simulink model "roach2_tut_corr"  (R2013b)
settings: Solver=VariableStepDiscrete  SolverMode=SingleTasking  StartTime=0.0  StopTime=100  RelTol=1e-3
undefined symbols (not defined in the file): add_latency, addr_width, Bit, bitfield, BitWidth, bram_latency, burst_size, casper_library_scopes, conv_latency, data_width, DelayLen, fan_latency, FFTSize, FFTStage, getfield, increment, led, Location, Lower, mult_latency, mux_latency, n_bits, n_bits_data, n_inputs, n_streams, n_taps, neg_latency, negate_latency, nsamples, pfb_size, pulse_len, reset_period, ROACH, ROACH2, snapshot, sx475t, sync_period, sync_period_bits, Upper, UseCounter, Width
libraries: xbsIndex_r4 x24444, casper_library_misc x73, xbsReplacements_r4 x34, casper_library_delays x14, xps_library x7
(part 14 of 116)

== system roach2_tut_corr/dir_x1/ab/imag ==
  addr : Inport
  data_in : Inport  Port=2
  we : Inport  Port=3
  calc_add : Subsystem
  convert_addr : xbsIndex_r4/Convert  gui_display_data_type=Fixed-point  arith_type=Unsigned  n_bits=addr_width  bin_pt=0  float_type=Single  exp_bits=8  fraction_bits=24  quantization=Truncate  overflow=Wrap  en=off  latency=0  dbl_ovrd=off  pipeline=off  block_type=convert
  convert_din1 : xbsIndex_r4/Convert  gui_display_data_type=Fixed-point  arith_type=Unsigned  n_bits=32  bin_pt=0  float_type=Single  exp_bits=8  fraction_bits=24  quantization=Truncate  overflow=Wrap  en=off  latency=0  dbl_ovrd=off  pipeline=off  block_type=convert
  convert_we : xbsIndex_r4/Convert  gui_display_data_type=Fixed-point  arith_type=Unsigned  n_bits=1  bin_pt=0  float_type=Single  exp_bits=8  fraction_bits=24  quantization=Truncate  overflow=Wrap  en=off  latency=0  dbl_ovrd=off  pipeline=off  block_type=convert
  mem : Subsystem
  munge_in : Subsystem  AncestorBlock=casper_library_flow_control/munge
  munge_out : Subsystem  AncestorBlock=casper_library_flow_control/munge
  roach2_tut_corr_dir_x1_ab_imag_addr : xbsIndex_r4/Gateway Out  inherit_from_input=off  hdl_port=on  timing_constraint=None  locs_specified=off  LOCs={'A5','B9','A9','C1','A3','G6','E9','A6','A7','A8','B8','B1','B3','D9','B5','B4','B6','C2'}  UseAsDAC=off  DACChannel='1'  block_type=gatewayout
  roach2_tut_corr_dir_x1_ab_imag_data_in : xbsIndex_r4/Gateway Out  inherit_from_input=off  hdl_port=on  timing_constraint=None  locs_specified=off  LOCs={'B21','B22','A22','B23','B19','C19','A20','A21','A23','B24','A24','A25','E18','D18','C18','B18'}  UseAsDAC=off  DACChannel='1'  block_type=gatewayout
  roach2_tut_corr_dir_x1_ab_imag_data_out : xbsIndex_r4/Gateway In  gui_display_data_type=Fixed-point  arith_type=Unsigned  n_bits=32  bin_pt=0  preci_type=Single  exp_width=8  frac_width=24  quantization=Truncate  overflow=Wrap  period=sample_rate  dbl_ovrd=off  timing_constraint=None  locs_specified=off  LOCs={}  UseAsADC=off  ADCChannel='1'  inherit_from_input=off  hdl_port=on  block_type=gatewayin
  roach2_tut_corr_dir_x1_ab_imag_we : xbsIndex_r4/Gateway Out  inherit_from_input=off  hdl_port=on  timing_constraint=None  locs_specified=off  LOCs={'A14'}  UseAsDAC=off  DACChannel='1'  block_type=gatewayout
  data_out : Outport
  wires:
  convert_addr/1 -> roach2_tut_corr_dir_x1_ab_imag_addr/1
  convert_din1/1 -> roach2_tut_corr_dir_x1_ab_imag_data_in/1
  data_in/1 -> munge_in/1(din)
  calc_add/1(out) -> convert_addr/1
  roach2_tut_corr_dir_x1_ab_imag_we/1 -> mem/3(In3)
  roach2_tut_corr_dir_x1_ab_imag_data_in/1 -> mem/2(In2)
  roach2_tut_corr_dir_x1_ab_imag_addr/1 -> mem/1(In1)
  convert_we/1 -> roach2_tut_corr_dir_x1_ab_imag_we/1
  roach2_tut_corr_dir_x1_ab_imag_data_out/1 -> munge_out/1(din)
  mem/1(Out1) -> roach2_tut_corr_dir_x1_ab_imag_data_out/1
  addr/1 -> calc_add/1(in)
  we/1 -> convert_we/1
  munge_out/1(dout) -> data_out/1
  munge_in/1(dout) -> convert_din1/1

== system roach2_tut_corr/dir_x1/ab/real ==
  addr : Inport
  data_in : Inport  Port=2
  we : Inport  Port=3
  calc_add : Subsystem
  convert_addr : xbsIndex_r4/Convert  gui_display_data_type=Fixed-point  arith_type=Unsigned  n_bits=addr_width  bin_pt=0  float_type=Single  exp_bits=8  fraction_bits=24  quantization=Truncate  overflow=Wrap  en=off  latency=0  dbl_ovrd=off  pipeline=off  block_type=convert
  convert_din1 : xbsIndex_r4/Convert  gui_display_data_type=Fixed-point  arith_type=Unsigned  n_bits=32  bin_pt=0  float_type=Single  exp_bits=8  fraction_bits=24  quantization=Truncate  overflow=Wrap  en=off  latency=0  dbl_ovrd=off  pipeline=off  block_type=convert
  convert_we : xbsIndex_r4/Convert  gui_display_data_type=Fixed-point  arith_type=Unsigned  n_bits=1  bin_pt=0  float_type=Single  exp_bits=8  fraction_bits=24  quantization=Truncate  overflow=Wrap  en=off  latency=0  dbl_ovrd=off  pipeline=off  block_type=convert
  mem : Subsystem
  munge_in : Subsystem  AncestorBlock=casper_library_flow_control/munge
  munge_out : Subsystem  AncestorBlock=casper_library_flow_control/munge
  roach2_tut_corr_dir_x1_ab_real_addr : xbsIndex_r4/Gateway Out  inherit_from_input=off  hdl_port=on  timing_constraint=None  locs_specified=off  LOCs={'A5','B9','A9','C1','A3','G6','E9','A6','A7','A8','B8','B1','B3','D9','B5','B4','B6','C2'}  UseAsDAC=off  DACChannel='1'  block_type=gatewayout
  roach2_tut_corr_dir_x1_ab_real_data_in : xbsIndex_r4/Gateway Out  inherit_from_input=off  hdl_port=on  timing_constraint=None  locs_specified=off  LOCs={'B21','B22','A22','B23','B19','C19','A20','A21','A23','B24','A24','A25','E18','D18','C18','B18'}  UseAsDAC=off  DACChannel='1'  block_type=gatewayout
  roach2_tut_corr_dir_x1_ab_real_data_out : xbsIndex_r4/Gateway In  gui_display_data_type=Fixed-point  arith_type=Unsigned  n_bits=32  bin_pt=0  preci_type=Single  exp_width=8  frac_width=24  quantization=Truncate  overflow=Wrap  period=sample_rate  dbl_ovrd=off  timing_constraint=None  locs_specified=off  LOCs={}  UseAsADC=off  ADCChannel='1'  inherit_from_input=off  hdl_port=on  block_type=gatewayin
  roach2_tut_corr_dir_x1_ab_real_we : xbsIndex_r4/Gateway Out  inherit_from_input=off  hdl_port=on  timing_constraint=None  locs_specified=off  LOCs={'A14'}  UseAsDAC=off  DACChannel='1'  block_type=gatewayout
  data_out : Outport
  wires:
  convert_addr/1 -> roach2_tut_corr_dir_x1_ab_real_addr/1
  convert_din1/1 -> roach2_tut_corr_dir_x1_ab_real_data_in/1
  data_in/1 -> munge_in/1(din)
  calc_add/1(out) -> convert_addr/1
  roach2_tut_corr_dir_x1_ab_real_we/1 -> mem/3(In3)
  roach2_tut_corr_dir_x1_ab_real_data_in/1 -> mem/2(In2)
  roach2_tut_corr_dir_x1_ab_real_addr/1 -> mem/1(In1)
  convert_we/1 -> roach2_tut_corr_dir_x1_ab_real_we/1
  roach2_tut_corr_dir_x1_ab_real_data_out/1 -> munge_out/1(din)
  mem/1(Out1) -> roach2_tut_corr_dir_x1_ab_real_data_out/1
  addr/1 -> calc_add/1(in)
  we/1 -> convert_we/1
  munge_out/1(dout) -> data_out/1
  munge_in/1(dout) -> convert_din1/1

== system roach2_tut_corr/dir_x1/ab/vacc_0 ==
  din : Inport
  new_acc : Inport  Port=2
  Adder0 : xbsIndex_r4/AddSub  mode=Addition  use_carryin=off  use_carryout=off  en=off  latency=2  precision=User Defined  arith_type="Signed  (2's comp)"  n_bits=32  bin_pt=6  quantization=Truncate  overflow=Wrap  dbl_ovrd=off  use_behavioral_HDL=on  hw_selection=Fabric  pipelined=off  use_rpm=on  block_type=addsub
  Mux0 : xbsIndex_r4/Mux  inputs=2  en=off  latency=0  precision=Full  arith_type="Signed  (2's comp)"  n_bits=8  bin_pt=2  quantization=Truncate  overflow=Wrap  dbl_ovrd=off  block_type=mux
  delay_bram : Subsystem
  pulse_ext : Subsystem
  warn period Adder00 : xbsReplacements_r4/Warning  period=1
  zero : xbsIndex_r4/Constant  const=0  gui_display_data_type=Fixed-point  arith_type=Signed (2's comp)  n_bits=32  bin_pt=6  preci_type=Single  exp_width=8  frac_width=24  explicit_period=on  period=1  equ=P=C  opselect=C  inp2=PCIN>>17  opr=+  inp1=P  carry=CIN  dbl_ovrd=off  block_type=constant
  dout : Outport
  valid : Outport  Port=2
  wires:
  delay_bram/1(Out1) -> Mux0/2, dout/1
  Adder0/1 -> delay_bram/1(In1)
  new_acc/1 -> pulse_ext/1(in)
  din/1 -> Adder0/1
  pulse_ext/1(out) -> valid/1, Mux0/1
  Mux0/1 -> Adder0/2
  zero/1 -> Mux0/3

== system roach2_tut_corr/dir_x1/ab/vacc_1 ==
  din : Inport
  new_acc : Inport  Port=2
  Adder0 : xbsIndex_r4/AddSub  mode=Addition  use_carryin=off  use_carryout=off  en=off  latency=2  precision=User Defined  arith_type="Signed  (2's comp)"  n_bits=32  bin_pt=6  quantization=Truncate  overflow=Wrap  dbl_ovrd=off  use_behavioral_HDL=on  hw_selection=Fabric  pipelined=off  use_rpm=on  block_type=addsub
  Mux0 : xbsIndex_r4/Mux  inputs=2  en=off  latency=0  precision=Full  arith_type="Signed  (2's comp)"  n_bits=8  bin_pt=2  quantization=Truncate  overflow=Wrap  dbl_ovrd=off  block_type=mux
  delay_bram : Subsystem
  pulse_ext : Subsystem
  warn period Adder00 : xbsReplacements_r4/Warning  period=1
  zero : xbsIndex_r4/Constant  const=0  gui_display_data_type=Fixed-point  arith_type=Signed (2's comp)  n_bits=32  bin_pt=6  preci_type=Single  exp_width=8  frac_width=24  explicit_period=on  period=1  equ=P=C  opselect=C  inp2=PCIN>>17  opr=+  inp1=P  carry=CIN  dbl_ovrd=off  block_type=constant
  dout : Outport
  valid : Outport  Port=2
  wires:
  zero/1 -> Mux0/3
  Mux0/1 -> Adder0/2
  pulse_ext/1(out) -> Mux0/1, valid/1
  din/1 -> Adder0/1
  new_acc/1 -> pulse_ext/1(in)
  Adder0/1 -> delay_bram/1(In1)
  delay_bram/1(Out1) -> dout/1, Mux0/2

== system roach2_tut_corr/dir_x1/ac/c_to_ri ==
  c : Inport
  force_im : xbsIndex_r4/Reinterpret  force_arith_type=on  arith_type="Signed  (2's comp)"  force_bin_pt=on  bin_pt=bin_pt  block_type=reinterpret
  force_re : xbsIndex_r4/Reinterpret  force_arith_type=on  arith_type="Signed  (2's comp)"  force_bin_pt=on  bin_pt=bin_pt  block_type=reinterpret
  slice_im : xbsIndex_r4/Slice  nbits=n_bits  boolean_output=off  mode=Lower Bit Location + Width  bit1=0  base1=MSB of Input  bit0=0  base0=LSB of Input  dbl_ovrd=off  block_type=slice
  slice_re : xbsIndex_r4/Slice  nbits=n_bits  boolean_output=off  mode=Upper Bit Location + Width  bit1=0  base1=MSB of Input  bit0=0  base0=LSB of Input  dbl_ovrd=off  block_type=slice
  re : Outport
  im : Outport  Port=2
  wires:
  c/1 -> slice_im/1, slice_re/1
  force_im/1 -> im/1
  force_re/1 -> re/1
  slice_im/1 -> force_im/1
  slice_re/1 -> force_re/1

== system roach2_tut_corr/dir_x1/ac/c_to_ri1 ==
  c : Inport
  force_im : xbsIndex_r4/Reinterpret  force_arith_type=on  arith_type="Signed  (2's comp)"  force_bin_pt=on  bin_pt=bin_pt  block_type=reinterpret
  force_re : xbsIndex_r4/Reinterpret  force_arith_type=on  arith_type="Signed  (2's comp)"  force_bin_pt=on  bin_pt=bin_pt  block_type=reinterpret
  slice_im : xbsIndex_r4/Slice  nbits=n_bits  boolean_output=off  mode=Lower Bit Location + Width  bit1=0  base1=MSB of Input  bit0=0  base0=LSB of Input  dbl_ovrd=off  block_type=slice
  slice_re : xbsIndex_r4/Slice  nbits=n_bits  boolean_output=off  mode=Upper Bit Location + Width  bit1=0  base1=MSB of Input  bit0=0  base0=LSB of Input  dbl_ovrd=off  block_type=slice
  re : Outport
  im : Outport  Port=2
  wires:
  c/1 -> slice_im/1, slice_re/1
  force_im/1 -> im/1
  force_re/1 -> re/1
  slice_im/1 -> force_im/1
  slice_re/1 -> force_re/1

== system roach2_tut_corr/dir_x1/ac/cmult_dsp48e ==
  a_re : Inport
  a_im : Inport  Port=2
  b_re : Inport  Port=3
  b_im : Inport  Port=4
  Convert{,1..2,5} (4 alike) : xbsIndex_r4/Convert  gui_display_data_type=Fixed-point  arith_type="Signed  (2's comp)"  n_bits=30  bin_pt=0  float_type=Single  exp_bits=8  fraction_bits=24  quantization=Truncate  overflow=Wrap  en=off  latency=0  dbl_ovrd=off  pipeline=on  block_type=convert
  Convert{3..4,6..7} (4 alike) : xbsIndex_r4/Convert  gui_display_data_type=Fixed-point  arith_type="Signed  (2's comp)"  n_bits=18  bin_pt=0  float_type=Single  exp_bits=8  fraction_bits=24  quantization=Truncate  overflow=Wrap  en=off  latency=0  dbl_ovrd=off  pipeline=on  block_type=convert
  DSP48E_0 : xbsIndex_r4/DSP48E  use_a=Direct from A Port  use_b=Direct from B Port  reset_preg=off  pattern_from_creg=off  pattern='000000000000'  mask_from_creg=off  pattern_mask='3FFFFFFFFFFF'  sel_rounding_mask=Select mask  use_op=off  use_creg=off  rst_all=off  en_all=off  use_pcin=off  use_carrycascin=off  use_multsignin=off  use_carryout=off  use_patterndetect=off  use_patternbdetect=off  use_overflow=off  use_underflow=off  use_acout=off  use_bcout=off  use_pcout=on  use_multsignout=off  use_carrycascout=off  pipeline_a=1  pipeline_b=1  pipeline_acout=1  pipeline_bcout=1  pipeline_c=on  pipeline_p=on  pipeline_mult=on  pipeline_opmode=on  pipeline_alumode=on  pipeline_carryin=on  pipeline_carryinsel=on  rst_a=off  rst_b=off  rst_c=off  rst_mult=off  rst_p=off  rst_carry_in=off  rst_alumode=off  rst_ctrl=off  en_a1=off  en_a2=off  en_b1=off  en_b2=off  en_c=off  en_mult=off  en_p=off  en_carry_in=off  en_alumode=off  en_multcarryin=off  en_ctrl=off  use_synth_model=off  addsub_mode=ONE48  xl_useadderonly=off  block_type=dsp48e
  DSP48E_1 : xbsIndex_r4/DSP48E  use_a=Direct from A Port  use_b=Direct from B Port  reset_preg=off  pattern_from_creg=off  pattern='000000000000'  mask_from_creg=off  pattern_mask='3FFFFFFFFFFF'  sel_rounding_mask=Select mask  use_op=off  use_creg=off  rst_all=off  en_all=off  use_pcin=on  use_carrycascin=off  use_multsignin=off  use_carryout=off  use_patterndetect=off  use_patternbdetect=off  use_overflow=off  use_underflow=off  use_acout=off  use_bcout=off  use_pcout=off  use_multsignout=off  use_carrycascout=off  pipeline_a=2  pipeline_b=2  pipeline_acout=1  pipeline_bcout=1  pipeline_c=on  pipeline_p=on  pipeline_mult=on  pipeline_opmode=on  pipeline_alumode=on  pipeline_carryin=on  pipeline_carryinsel=on  rst_a=off  rst_b=off  rst_c=off  rst_mult=off  rst_p=off  rst_carry_in=off  rst_alumode=off  rst_ctrl=off  en_a1=off  en_a2=off  en_b1=off  en_b2=off  en_c=off  en_mult=off  en_p=off  en_carry_in=off  en_alumode=off  en_multcarryin=off  en_ctrl=off  use_synth_model=off  addsub_mode=ONE48  xl_useadderonly=off  block_type=dsp48e
  DSP48E_2 : xbsIndex_r4/DSP48E  use_a=Direct from A Port  use_b=Direct from B Port  reset_preg=off  pattern_from_creg=off  pattern='000000000000'  mask_from_creg=off  pattern_mask='3FFFFFFFFFFF'  sel_rounding_mask=Select mask  use_op=off  use_creg=off  rst_all=off  en_all=off  use_pcin=off  use_carrycascin=off  use_multsignin=off  use_carryout=off  use_patterndetect=off  use_patternbdetect=off  use_overflow=off  use_underflow=off  use_acout=off  use_bcout=off  use_pcout=on  use_multsignout=off  use_carrycascout=off  pipeline_a=1  pipeline_b=1  pipeline_acout=1  pipeline_bcout=1  pipeline_c=on  pipeline_p=on  pipeline_mult=on  pipeline_opmode=on  pipeline_alumode=on  pipeline_carryin=on  pipeline_carryinsel=on  rst_a=off  rst_b=off  rst_c=off  rst_mult=off  rst_p=off  rst_carry_in=off  rst_alumode=off  rst_ctrl=off  en_a1=off  en_a2=off  en_b1=off  en_b2=off  en_c=off  en_mult=off  en_p=off  en_carry_in=off  en_alumode=off  en_multcarryin=off  en_ctrl=off  use_synth_model=off  addsub_mode=ONE48  xl_useadderonly=off  block_type=dsp48e
  DSP48E_3 : xbsIndex_r4/DSP48E  use_a=Direct from A Port  use_b=Direct from B Port  reset_preg=off  pattern_from_creg=off  pattern='000000000000'  mask_from_creg=off  pattern_mask='3FFFFFFFFFFF'  sel_rounding_mask=Select mask  use_op=off  use_creg=off  rst_all=off  en_all=off  use_pcin=on  use_carrycascin=off  use_multsignin=off  use_carryout=off  use_patterndetect=off  use_patternbdetect=off  use_overflow=off  use_underflow=off  use_acout=off  use_bcout=off  use_pcout=off  use_multsignout=off  use_carrycascout=off  pipeline_a=2  pipeline_b=2  pipeline_acout=1  pipeline_bcout=1  pipeline_c=on  pipeline_p=on  pipeline_mult=on  pipeline_opmode=on  pipeline_alumode=on  pipeline_carryin=on  pipeline_carryinsel=on  rst_a=off  rst_b=off  rst_c=off  rst_mult=off  rst_p=off  rst_carry_in=off  rst_alumode=off  rst_ctrl=off  en_a1=off  en_a2=off  en_b1=off  en_b2=off  en_c=off  en_mult=off  en_p=off  en_carry_in=off  en_alumode=off  en_multcarryin=off  en_ctrl=off  use_synth_model=off  addsub_mode=ONE48  xl_useadderonly=off  block_type=dsp48e
  Terminator : Terminator
  Terminator1 : Terminator
  alumode0 : xbsIndex_r4/Constant  const=3  gui_display_data_type=Fixed-point  arith_type=Unsigned  n_bits=4  bin_pt=0  preci_type=Single  exp_width=8  frac_width=24  explicit_period=off  period=1  equ=P=C  opselect=C  inp2=PCIN>>17  opr=+  inp1=P  carry=CIN  dbl_ovrd=off  block_type=constant
  alumode1 : xbsIndex_r4/Constant  const=0  gui_display_data_type=Fixed-point  arith_type=Unsigned  n_bits=4  bin_pt=0  preci_type=Single  exp_width=8  frac_width=24  explicit_period=off  period=1  equ=P=C  opselect=C  inp2=PCIN>>17  opr=+  inp1=P  carry=CIN  dbl_ovrd=off  block_type=constant
  alumode2 : xbsIndex_r4/Constant  const=0  gui_display_data_type=Fixed-point  arith_type=Unsigned  n_bits=4  bin_pt=0  preci_type=Single  exp_width=8  frac_width=24  explicit_period=off  period=1  equ=P=C  opselect=C  inp2=PCIN>>17  opr=+  inp1=P  carry=CIN  dbl_ovrd=off  block_type=constant
  alumode3 : xbsIndex_r4/Constant  const=0  gui_display_data_type=Fixed-point  arith_type=Unsigned  n_bits=4  bin_pt=0  preci_type=Single  exp_width=8  frac_width=24  explicit_period=off  period=1  equ=P=C  opselect=C  inp2=PCIN>>17  opr=+  inp1=P  carry=CIN  dbl_ovrd=off  block_type=constant
  carryin{0..3} (4 alike) : xbsIndex_r4/Constant  const=0  gui_display_data_type=Fixed-point  arith_type=Unsigned  n_bits=1  bin_pt=0  preci_type=Single  exp_width=8  frac_width=24  explicit_period=off  period=1  equ=P=C  opselect=C  inp2=PCIN>>17  opr=+  inp1=P  carry=CIN  dbl_ovrd=off  block_type=constant
  carryinsel{0..3} (4 alike) : xbsIndex_r4/Constant  const=0  gui_display_data_type=Fixed-point  arith_type=Unsigned  n_bits=3  bin_pt=0  preci_type=Single  exp_width=8  frac_width=24  explicit_period=off  period=1  equ=P=C  opselect=C  inp2=PCIN>>17  opr=+  inp1=P  carry=CIN  dbl_ovrd=off  block_type=constant
  cast_c_im : xbsIndex_r4/Convert  gui_display_data_type=Fixed-point  arith_type="Signed  (2's comp)"  n_bits=9  bin_pt=6  float_type=Single  exp_bits=8  fraction_bits=24  quantization=Truncate  overflow=Wrap  en=off  latency=0  dbl_ovrd=off  pipeline=on  block_type=convert
  cast_c_re : xbsIndex_r4/Convert  gui_display_data_type=Fixed-point  arith_type="Signed  (2's comp)"  n_bits=9  bin_pt=6  float_type=Single  exp_bits=8  fraction_bits=24  quantization=Truncate  overflow=Wrap  en=off  latency=0  dbl_ovrd=off  pipeline=on  block_type=convert
  opmode0 : xbsIndex_r4/Constant  const=5  gui_display_data_type=Fixed-point  arith_type=Unsigned  n_bits=7  bin_pt=0  preci_type=Single  exp_width=8  frac_width=24  explicit_period=off  period=1  equ=P=C  opselect=C  inp2=PCIN>>17  opr=+  inp1=P  carry=CIN  dbl_ovrd=off  block_type=constant
  opmode1 : xbsIndex_r4/Constant  const=21  gui_display_data_type=Fixed-point  arith_type=Unsigned  n_bits=7  bin_pt=0  preci_type=Single  exp_width=8  frac_width=24  explicit_period=off  period=1  equ=P=C  opselect=C  inp2=PCIN>>17  opr=+  inp1=P  carry=CIN  dbl_ovrd=off  block_type=constant
  opmode2 : xbsIndex_r4/Constant  const=5  gui_display_data_type=Fixed-point  arith_type=Unsigned  n_bits=7  bin_pt=0  preci_type=Single  exp_width=8  frac_width=24  explicit_period=off  period=1  equ=P=C  opselect=C  inp2=PCIN>>17  opr=+  inp1=P  carry=CIN  dbl_ovrd=off  block_type=constant
  opmode3 : xbsIndex_r4/Constant  const=21  gui_display_data_type=Fixed-point  arith_type=Unsigned  n_bits=7  bin_pt=0  preci_type=Single  exp_width=8  frac_width=24  explicit_period=off  period=1  equ=P=C  opselect=C  inp2=PCIN>>17  opr=+  inp1=P  carry=CIN  dbl_ovrd=off  block_type=constant
  realign_a_im : xbsIndex_r4/Convert  gui_display_data_type=Fixed-point  arith_type="Signed  (2's comp)"  n_bits=4  bin_pt=3  float_type=Single  exp_bits=8  fraction_bits=24  quantization=Truncate  overflow=Wrap  en=off  latency=0  dbl_ovrd=off  pipeline=on  block_type=convert
  realign_a_re : xbsIndex_r4/Convert  gui_display_data_type=Fixed-point  arith_type="Signed  (2's comp)"  n_bits=4  bin_pt=3  float_type=Single  exp_bits=8  fraction_bits=24  quantization=Truncate  overflow=Wrap  en=off  latency=0  dbl_ovrd=off  pipeline=on  block_type=convert
  realign_b_im : xbsIndex_r4/Convert  gui_display_data_type=Fixed-point  arith_type="Signed  (2's comp)"  n_bits=4  bin_pt=3  float_type=Single  exp_bits=8  fraction_bits=24  quantization=Truncate  overflow=Wrap  en=off  latency=0  dbl_ovrd=off  pipeline=on  block_type=convert
  realign_b_re : xbsIndex_r4/Convert  gui_display_data_type=Fixed-point  arith_type="Signed  (2's comp)"  n_bits=4  bin_pt=3  float_type=Single  exp_bits=8  fraction_bits=24  quantization=Truncate  overflow=Wrap  en=off  latency=0  dbl_ovrd=off  pipeline=on  block_type=convert
  reinterp_a_im : xbsIndex_r4/Reinterpret  force_arith_type=on  arith_type="Signed  (2's comp)"  force_bin_pt=on  bin_pt=0  block_type=reinterpret
  reinterp_a_re : xbsIndex_r4/Reinterpret  force_arith_type=on  arith_type="Signed  (2's comp)"  force_bin_pt=on  bin_pt=0  block_type=reinterpret
  reinterp_b_im : xbsIndex_r4/Reinterpret  force_arith_type=on  arith_type="Signed  (2's comp)"  force_bin_pt=on  bin_pt=0  block_type=reinterpret
  reinterp_b_re : xbsIndex_r4/Reinterpret  force_arith_type=on  arith_type="Signed  (2's comp)"  force_bin_pt=on  bin_pt=0  block_type=reinterpret
  reinterp_c_im : xbsIndex_r4/Reinterpret  force_arith_type=on  arith_type="Signed  (2's comp)"  force_bin_pt=on  bin_pt=6  block_type=reinterpret
  reinterp_c_re : xbsIndex_r4/Reinterpret  force_arith_type=on  arith_type="Signed  (2's comp)"  force_bin_pt=on  bin_pt=6  block_type=reinterpret
  c_re : Outport
  c_im : Outport  Port=2
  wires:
  b_im/1 -> realign_b_im/1
  b_re/1 -> realign_b_re/1
  a_im/1 -> realign_a_im/1
  a_re/1 -> realign_a_re/1
  cast_c_im/1 -> c_im/1
  cast_c_re/1 -> c_re/1
  reinterp_b_im/1 -> Convert3/1, Convert7/1
  reinterp_b_re/1 -> Convert6/1, Convert4/1
  reinterp_a_im/1 -> Convert/1, Convert1/1
  reinterp_a_re/1 -> Convert5/1, Convert2/1
  realign_b_im/1 -> reinterp_b_im/1
  realign_b_re/1 -> reinterp_b_re/1
  realign_a_im/1 -> reinterp_a_im/1
  realign_a_re/1 -> reinterp_a_re/1
  Convert/1 -> DSP48E_3/1
  DSP48E_2/1 -> Terminator/1
  DSP48E_2/2 -> DSP48E_3/3
  opmode3/1 -> DSP48E_3/4
  alumode3/1 -> DSP48E_3/5
  carryin3/1 -> DSP48E_3/6
  carryinsel3/1 -> DSP48E_3/7
  Convert3/1 -> DSP48E_3/2
  Convert2/1 -> DSP48E_2/1
  Convert4/1 -> DSP48E_2/2
  opmode2/1 -> DSP48E_2/3
  alumode2/1 -> DSP48E_2/4
  carryin2/1 -> DSP48E_2/5
  carryinsel2/1 -> DSP48E_2/6
  reinterp_c_re/1 -> cast_c_re/1
  DSP48E_3/1 -> reinterp_c_re/1
  Convert1/1 -> DSP48E_1/1
  DSP48E_0/1 -> Terminator1/1
  DSP48E_0/2 -> DSP48E_1/3
  opmode1/1 -> DSP48E_1/4
  alumode1/1 -> DSP48E_1/5
  carryin1/1 -> DSP48E_1/6
  carryinsel1/1 -> DSP48E_1/7
  Convert6/1 -> DSP48E_1/2
  Convert5/1 -> DSP48E_0/1
  Convert7/1 -> DSP48E_0/2
  opmode0/1 -> DSP48E_0/3
  alumode0/1 -> DSP48E_0/4
  carryin0/1 -> DSP48E_0/5
  carryinsel0/1 -> DSP48E_0/6
  DSP48E_1/1 -> reinterp_c_im/1
  reinterp_c_im/1 -> cast_c_im/1

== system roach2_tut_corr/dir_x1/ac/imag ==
  addr : Inport
  data_in : Inport  Port=2
  we : Inport  Port=3
  calc_add : Subsystem
  convert_addr : xbsIndex_r4/Convert  gui_display_data_type=Fixed-point  arith_type=Unsigned  n_bits=addr_width  bin_pt=0  float_type=Single  exp_bits=8  fraction_bits=24  quantization=Truncate  overflow=Wrap  en=off  latency=0  dbl_ovrd=off  pipeline=off  block_type=convert
  convert_din1 : xbsIndex_r4/Convert  gui_display_data_type=Fixed-point  arith_type=Unsigned  n_bits=32  bin_pt=0  float_type=Single  exp_bits=8  fraction_bits=24  quantization=Truncate  overflow=Wrap  en=off  latency=0  dbl_ovrd=off  pipeline=off  block_type=convert
  convert_we : xbsIndex_r4/Convert  gui_display_data_type=Fixed-point  arith_type=Unsigned  n_bits=1  bin_pt=0  float_type=Single  exp_bits=8  fraction_bits=24  quantization=Truncate  overflow=Wrap  en=off  latency=0  dbl_ovrd=off  pipeline=off  block_type=convert
  mem : Subsystem
  munge_in : Subsystem  AncestorBlock=casper_library_flow_control/munge
  munge_out : Subsystem  AncestorBlock=casper_library_flow_control/munge
  roach2_tut_corr_dir_x1_ac_imag_addr : xbsIndex_r4/Gateway Out  inherit_from_input=off  hdl_port=on  timing_constraint=None  locs_specified=off  LOCs={'A5','B9','A9','C1','A3','G6','E9','A6','A7','A8','B8','B1','B3','D9','B5','B4','B6','C2'}  UseAsDAC=off  DACChannel='1'  block_type=gatewayout
  roach2_tut_corr_dir_x1_ac_imag_data_in : xbsIndex_r4/Gateway Out  inherit_from_input=off  hdl_port=on  timing_constraint=None  locs_specified=off  LOCs={'B21','B22','A22','B23','B19','C19','A20','A21','A23','B24','A24','A25','E18','D18','C18','B18'}  UseAsDAC=off  DACChannel='1'  block_type=gatewayout
  roach2_tut_corr_dir_x1_ac_imag_data_out : xbsIndex_r4/Gateway In  gui_display_data_type=Fixed-point  arith_type=Unsigned  n_bits=32  bin_pt=0  preci_type=Single  exp_width=8  frac_width=24  quantization=Truncate  overflow=Wrap  period=sample_rate  dbl_ovrd=off  timing_constraint=None  locs_specified=off  LOCs={}  UseAsADC=off  ADCChannel='1'  inherit_from_input=off  hdl_port=on  block_type=gatewayin
  roach2_tut_corr_dir_x1_ac_imag_we : xbsIndex_r4/Gateway Out  inherit_from_input=off  hdl_port=on  timing_constraint=None  locs_specified=off  LOCs={'A14'}  UseAsDAC=off  DACChannel='1'  block_type=gatewayout
  data_out : Outport
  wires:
  convert_addr/1 -> roach2_tut_corr_dir_x1_ac_imag_addr/1
  convert_din1/1 -> roach2_tut_corr_dir_x1_ac_imag_data_in/1
  data_in/1 -> munge_in/1(din)
  calc_add/1(out) -> convert_addr/1
  roach2_tut_corr_dir_x1_ac_imag_we/1 -> mem/3(In3)
  roach2_tut_corr_dir_x1_ac_imag_data_in/1 -> mem/2(In2)
  roach2_tut_corr_dir_x1_ac_imag_addr/1 -> mem/1(In1)
  convert_we/1 -> roach2_tut_corr_dir_x1_ac_imag_we/1
  roach2_tut_corr_dir_x1_ac_imag_data_out/1 -> munge_out/1(din)
  mem/1(Out1) -> roach2_tut_corr_dir_x1_ac_imag_data_out/1
  addr/1 -> calc_add/1(in)
  we/1 -> convert_we/1
  munge_out/1(dout) -> data_out/1
  munge_in/1(dout) -> convert_din1/1

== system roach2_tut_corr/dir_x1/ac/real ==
  addr : Inport
  data_in : Inport  Port=2
  we : Inport  Port=3
  calc_add : Subsystem
  convert_addr : xbsIndex_r4/Convert  gui_display_data_type=Fixed-point  arith_type=Unsigned  n_bits=addr_width  bin_pt=0  float_type=Single  exp_bits=8  fraction_bits=24  quantization=Truncate  overflow=Wrap  en=off  latency=0  dbl_ovrd=off  pipeline=off  block_type=convert
  convert_din1 : xbsIndex_r4/Convert  gui_display_data_type=Fixed-point  arith_type=Unsigned  n_bits=32  bin_pt=0  float_type=Single  exp_bits=8  fraction_bits=24  quantization=Truncate  overflow=Wrap  en=off  latency=0  dbl_ovrd=off  pipeline=off  block_type=convert
  convert_we : xbsIndex_r4/Convert  gui_display_data_type=Fixed-point  arith_type=Unsigned  n_bits=1  bin_pt=0  float_type=Single  exp_bits=8  fraction_bits=24  quantization=Truncate  overflow=Wrap  en=off  latency=0  dbl_ovrd=off  pipeline=off  block_type=convert
  mem : Subsystem
  munge_in : Subsystem  AncestorBlock=casper_library_flow_control/munge
  munge_out : Subsystem  AncestorBlock=casper_library_flow_control/munge
  roach2_tut_corr_dir_x1_ac_real_addr : xbsIndex_r4/Gateway Out  inherit_from_input=off  hdl_port=on  timing_constraint=None  locs_specified=off  LOCs={'A5','B9','A9','C1','A3','G6','E9','A6','A7','A8','B8','B1','B3','D9','B5','B4','B6','C2'}  UseAsDAC=off  DACChannel='1'  block_type=gatewayout
  roach2_tut_corr_dir_x1_ac_real_data_in : xbsIndex_r4/Gateway Out  inherit_from_input=off  hdl_port=on  timing_constraint=None  locs_specified=off  LOCs={'B21','B22','A22','B23','B19','C19','A20','A21','A23','B24','A24','A25','E18','D18','C18','B18'}  UseAsDAC=off  DACChannel='1'  block_type=gatewayout
  roach2_tut_corr_dir_x1_ac_real_data_out : xbsIndex_r4/Gateway In  gui_display_data_type=Fixed-point  arith_type=Unsigned  n_bits=32  bin_pt=0  preci_type=Single  exp_width=8  frac_width=24  quantization=Truncate  overflow=Wrap  period=sample_rate  dbl_ovrd=off  timing_constraint=None  locs_specified=off  LOCs={}  UseAsADC=off  ADCChannel='1'  inherit_from_input=off  hdl_port=on  block_type=gatewayin
  roach2_tut_corr_dir_x1_ac_real_we : xbsIndex_r4/Gateway Out  inherit_from_input=off  hdl_port=on  timing_constraint=None  locs_specified=off  LOCs={'A14'}  UseAsDAC=off  DACChannel='1'  block_type=gatewayout
  data_out : Outport
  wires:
  convert_addr/1 -> roach2_tut_corr_dir_x1_ac_real_addr/1
  convert_din1/1 -> roach2_tut_corr_dir_x1_ac_real_data_in/1
  data_in/1 -> munge_in/1(din)
  calc_add/1(out) -> convert_addr/1
  roach2_tut_corr_dir_x1_ac_real_we/1 -> mem/3(In3)
  roach2_tut_corr_dir_x1_ac_real_data_in/1 -> mem/2(In2)
  roach2_tut_corr_dir_x1_ac_real_addr/1 -> mem/1(In1)
  convert_we/1 -> roach2_tut_corr_dir_x1_ac_real_we/1
  roach2_tut_corr_dir_x1_ac_real_data_out/1 -> munge_out/1(din)
  mem/1(Out1) -> roach2_tut_corr_dir_x1_ac_real_data_out/1
  addr/1 -> calc_add/1(in)
  we/1 -> convert_we/1
  munge_out/1(dout) -> data_out/1
  munge_in/1(dout) -> convert_din1/1

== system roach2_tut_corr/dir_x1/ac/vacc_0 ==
  din : Inport
  new_acc : Inport  Port=2
  Adder0 : xbsIndex_r4/AddSub  mode=Addition  use_carryin=off  use_carryout=off  en=off  latency=2  precision=User Defined  arith_type="Signed  (2's comp)"  n_bits=32  bin_pt=6  quantization=Truncate  overflow=Wrap  dbl_ovrd=off  use_behavioral_HDL=on  hw_selection=Fabric  pipelined=off  use_rpm=on  block_type=addsub
  Mux0 : xbsIndex_r4/Mux  inputs=2  en=off  latency=0  precision=Full  arith_type="Signed  (2's comp)"  n_bits=8  bin_pt=2  quantization=Truncate  overflow=Wrap  dbl_ovrd=off  block_type=mux
  delay_bram : Subsystem
  pulse_ext : Subsystem
  warn period Adder00 : xbsReplacements_r4/Warning  period=1
  zero : xbsIndex_r4/Constant  const=0  gui_display_data_type=Fixed-point  arith_type=Signed (2's comp)  n_bits=32  bin_pt=6  preci_type=Single  exp_width=8  frac_width=24  explicit_period=on  period=1  equ=P=C  opselect=C  inp2=PCIN>>17  opr=+  inp1=P  carry=CIN  dbl_ovrd=off  block_type=constant
  dout : Outport
  valid : Outport  Port=2
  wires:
  zero/1 -> Mux0/3
  Mux0/1 -> Adder0/2
  pulse_ext/1(out) -> Mux0/1, valid/1
  din/1 -> Adder0/1
  new_acc/1 -> pulse_ext/1(in)
  Adder0/1 -> delay_bram/1(In1)
  delay_bram/1(Out1) -> dout/1, Mux0/2

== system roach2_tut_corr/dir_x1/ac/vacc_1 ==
  din : Inport
  new_acc : Inport  Port=2
  Adder0 : xbsIndex_r4/AddSub  mode=Addition  use_carryin=off  use_carryout=off  en=off  latency=2  precision=User Defined  arith_type="Signed  (2's comp)"  n_bits=32  bin_pt=6  quantization=Truncate  overflow=Wrap  dbl_ovrd=off  use_behavioral_HDL=on  hw_selection=Fabric  pipelined=off  use_rpm=on  block_type=addsub
  Mux0 : xbsIndex_r4/Mux  inputs=2  en=off  latency=0  precision=Full  arith_type="Signed  (2's comp)"  n_bits=8  bin_pt=2  quantization=Truncate  overflow=Wrap  dbl_ovrd=off  block_type=mux
  delay_bram : Subsystem
  pulse_ext : Subsystem
  warn period Adder00 : xbsReplacements_r4/Warning  period=1
  zero : xbsIndex_r4/Constant  const=0  gui_display_data_type=Fixed-point  arith_type=Signed (2's comp)  n_bits=32  bin_pt=6  preci_type=Single  exp_width=8  frac_width=24  explicit_period=on  period=1  equ=P=C  opselect=C  inp2=PCIN>>17  opr=+  inp1=P  carry=CIN  dbl_ovrd=off  block_type=constant
  dout : Outport
  valid : Outport  Port=2
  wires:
  delay_bram/1(Out1) -> Mux0/2, dout/1
  Adder0/1 -> delay_bram/1(In1)
  new_acc/1 -> pulse_ext/1(in)
  din/1 -> Adder0/1
  pulse_ext/1(out) -> valid/1, Mux0/1
  Mux0/1 -> Adder0/2
  zero/1 -> Mux0/3

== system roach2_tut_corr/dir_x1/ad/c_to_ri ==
  c : Inport
  force_im : xbsIndex_r4/Reinterpret  force_arith_type=on  arith_type="Signed  (2's comp)"  force_bin_pt=on  bin_pt=bin_pt  block_type=reinterpret
  force_re : xbsIndex_r4/Reinterpret  force_arith_type=on  arith_type="Signed  (2's comp)"  force_bin_pt=on  bin_pt=bin_pt  block_type=reinterpret
  slice_im : xbsIndex_r4/Slice  nbits=n_bits  boolean_output=off  mode=Lower Bit Location + Width  bit1=0  base1=MSB of Input  bit0=0  base0=LSB of Input  dbl_ovrd=off  block_type=slice
  slice_re : xbsIndex_r4/Slice  nbits=n_bits  boolean_output=off  mode=Upper Bit Location + Width  bit1=0  base1=MSB of Input  bit0=0  base0=LSB of Input  dbl_ovrd=off  block_type=slice
  re : Outport
  im : Outport  Port=2
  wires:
  slice_re/1 -> force_re/1
  slice_im/1 -> force_im/1
  force_re/1 -> re/1
  force_im/1 -> im/1
  c/1 -> slice_re/1, slice_im/1

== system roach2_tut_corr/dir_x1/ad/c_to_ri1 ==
  c : Inport
  force_im : xbsIndex_r4/Reinterpret  force_arith_type=on  arith_type="Signed  (2's comp)"  force_bin_pt=on  bin_pt=bin_pt  block_type=reinterpret
  force_re : xbsIndex_r4/Reinterpret  force_arith_type=on  arith_type="Signed  (2's comp)"  force_bin_pt=on  bin_pt=bin_pt  block_type=reinterpret
  slice_im : xbsIndex_r4/Slice  nbits=n_bits  boolean_output=off  mode=Lower Bit Location + Width  bit1=0  base1=MSB of Input  bit0=0  base0=LSB of Input  dbl_ovrd=off  block_type=slice
  slice_re : xbsIndex_r4/Slice  nbits=n_bits  boolean_output=off  mode=Upper Bit Location + Width  bit1=0  base1=MSB of Input  bit0=0  base0=LSB of Input  dbl_ovrd=off  block_type=slice
  re : Outport
  im : Outport  Port=2
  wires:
  slice_re/1 -> force_re/1
  slice_im/1 -> force_im/1
  force_re/1 -> re/1
  force_im/1 -> im/1
  c/1 -> slice_re/1, slice_im/1

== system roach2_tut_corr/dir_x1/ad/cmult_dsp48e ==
  a_re : Inport
  a_im : Inport  Port=2
  b_re : Inport  Port=3
  b_im : Inport  Port=4
  Convert{,1..2,5} (4 alike) : xbsIndex_r4/Convert  gui_display_data_type=Fixed-point  arith_type="Signed  (2's comp)"  n_bits=30  bin_pt=0  float_type=Single  exp_bits=8  fraction_bits=24  quantization=Truncate  overflow=Wrap  en=off  latency=0  dbl_ovrd=off  pipeline=on  block_type=convert
  Convert{3..4,6..7} (4 alike) : xbsIndex_r4/Convert  gui_display_data_type=Fixed-point  arith_type="Signed  (2's comp)"  n_bits=18  bin_pt=0  float_type=Single  exp_bits=8  fraction_bits=24  quantization=Truncate  overflow=Wrap  en=off  latency=0  dbl_ovrd=off  pipeline=on  block_type=convert
  DSP48E_0 : xbsIndex_r4/DSP48E  use_a=Direct from A Port  use_b=Direct from B Port  reset_preg=off  pattern_from_creg=off  pattern='000000000000'  mask_from_creg=off  pattern_mask='3FFFFFFFFFFF'  sel_rounding_mask=Select mask  use_op=off  use_creg=off  rst_all=off  en_all=off  use_pcin=off  use_carrycascin=off  use_multsignin=off  use_carryout=off  use_patterndetect=off  use_patternbdetect=off  use_overflow=off  use_underflow=off  use_acout=off  use_bcout=off  use_pcout=on  use_multsignout=off  use_carrycascout=off  pipeline_a=1  pipeline_b=1  pipeline_acout=1  pipeline_bcout=1  pipeline_c=on  pipeline_p=on  pipeline_mult=on  pipeline_opmode=on  pipeline_alumode=on  pipeline_carryin=on  pipeline_carryinsel=on  rst_a=off  rst_b=off  rst_c=off  rst_mult=off  rst_p=off  rst_carry_in=off  rst_alumode=off  rst_ctrl=off  en_a1=off  en_a2=off  en_b1=off  en_b2=off  en_c=off  en_mult=off  en_p=off  en_carry_in=off  en_alumode=off  en_multcarryin=off  en_ctrl=off  use_synth_model=off  addsub_mode=ONE48  xl_useadderonly=off  block_type=dsp48e
  DSP48E_1 : xbsIndex_r4/DSP48E  use_a=Direct from A Port  use_b=Direct from B Port  reset_preg=off  pattern_from_creg=off  pattern='000000000000'  mask_from_creg=off  pattern_mask='3FFFFFFFFFFF'  sel_rounding_mask=Select mask  use_op=off  use_creg=off  rst_all=off  en_all=off  use_pcin=on  use_carrycascin=off  use_multsignin=off  use_carryout=off  use_patterndetect=off  use_patternbdetect=off  use_overflow=off  use_underflow=off  use_acout=off  use_bcout=off  use_pcout=off  use_multsignout=off  use_carrycascout=off  pipeline_a=2  pipeline_b=2  pipeline_acout=1  pipeline_bcout=1  pipeline_c=on  pipeline_p=on  pipeline_mult=on  pipeline_opmode=on  pipeline_alumode=on  pipeline_carryin=on  pipeline_carryinsel=on  rst_a=off  rst_b=off  rst_c=off  rst_mult=off  rst_p=off  rst_carry_in=off  rst_alumode=off  rst_ctrl=off  en_a1=off  en_a2=off  en_b1=off  en_b2=off  en_c=off  en_mult=off  en_p=off  en_carry_in=off  en_alumode=off  en_multcarryin=off  en_ctrl=off  use_synth_model=off  addsub_mode=ONE48  xl_useadderonly=off  block_type=dsp48e
  DSP48E_2 : xbsIndex_r4/DSP48E  use_a=Direct from A Port  use_b=Direct from B Port  reset_preg=off  pattern_from_creg=off  pattern='000000000000'  mask_from_creg=off  pattern_mask='3FFFFFFFFFFF'  sel_rounding_mask=Select mask  use_op=off  use_creg=off  rst_all=off  en_all=off  use_pcin=off  use_carrycascin=off  use_multsignin=off  use_carryout=off  use_patterndetect=off  use_patternbdetect=off  use_overflow=off  use_underflow=off  use_acout=off  use_bcout=off  use_pcout=on  use_multsignout=off  use_carrycascout=off  pipeline_a=1  pipeline_b=1  pipeline_acout=1  pipeline_bcout=1  pipeline_c=on  pipeline_p=on  pipeline_mult=on  pipeline_opmode=on  pipeline_alumode=on  pipeline_carryin=on  pipeline_carryinsel=on  rst_a=off  rst_b=off  rst_c=off  rst_mult=off  rst_p=off  rst_carry_in=off  rst_alumode=off  rst_ctrl=off  en_a1=off  en_a2=off  en_b1=off  en_b2=off  en_c=off  en_mult=off  en_p=off  en_carry_in=off  en_alumode=off  en_multcarryin=off  en_ctrl=off  use_synth_model=off  addsub_mode=ONE48  xl_useadderonly=off  block_type=dsp48e
  DSP48E_3 : xbsIndex_r4/DSP48E  use_a=Direct from A Port  use_b=Direct from B Port  reset_preg=off  pattern_from_creg=off  pattern='000000000000'  mask_from_creg=off  pattern_mask='3FFFFFFFFFFF'  sel_rounding_mask=Select mask  use_op=off  use_creg=off  rst_all=off  en_all=off  use_pcin=on  use_carrycascin=off  use_multsignin=off  use_carryout=off  use_patterndetect=off  use_patternbdetect=off  use_overflow=off  use_underflow=off  use_acout=off  use_bcout=off  use_pcout=off  use_multsignout=off  use_carrycascout=off  pipeline_a=2  pipeline_b=2  pipeline_acout=1  pipeline_bcout=1  pipeline_c=on  pipeline_p=on  pipeline_mult=on  pipeline_opmode=on  pipeline_alumode=on  pipeline_carryin=on  pipeline_carryinsel=on  rst_a=off  rst_b=off  rst_c=off  rst_mult=off  rst_p=off  rst_carry_in=off  rst_alumode=off  rst_ctrl=off  en_a1=off  en_a2=off  en_b1=off  en_b2=off  en_c=off  en_mult=off  en_p=off  en_carry_in=off  en_alumode=off  en_multcarryin=off  en_ctrl=off  use_synth_model=off  addsub_mode=ONE48  xl_useadderonly=off  block_type=dsp48e
  Terminator : Terminator
  Terminator1 : Terminator
  alumode0 : xbsIndex_r4/Constant  const=3  gui_display_data_type=Fixed-point  arith_type=Unsigned  n_bits=4  bin_pt=0  preci_type=Single  exp_width=8  frac_width=24  explicit_period=off  period=1  equ=P=C  opselect=C  inp2=PCIN>>17  opr=+  inp1=P  carry=CIN  dbl_ovrd=off  block_type=constant
  alumode1 : xbsIndex_r4/Constant  const=0  gui_display_data_type=Fixed-point  arith_type=Unsigned  n_bits=4  bin_pt=0  preci_type=Single  exp_width=8  frac_width=24  explicit_period=off  period=1  equ=P=C  opselect=C  inp2=PCIN>>17  opr=+  inp1=P  carry=CIN  dbl_ovrd=off  block_type=constant
  alumode2 : xbsIndex_r4/Constant  const=0  gui_display_data_type=Fixed-point  arith_type=Unsigned  n_bits=4  bin_pt=0  preci_type=Single  exp_width=8  frac_width=24  explicit_period=off  period=1  equ=P=C  opselect=C  inp2=PCIN>>17  opr=+  inp1=P  carry=CIN  dbl_ovrd=off  block_type=constant
  alumode3 : xbsIndex_r4/Constant  const=0  gui_display_data_type=Fixed-point  arith_type=Unsigned  n_bits=4  bin_pt=0  preci_type=Single  exp_width=8  frac_width=24  explicit_period=off  period=1  equ=P=C  opselect=C  inp2=PCIN>>17  opr=+  inp1=P  carry=CIN  dbl_ovrd=off  block_type=constant
  carryin{0..3} (4 alike) : xbsIndex_r4/Constant  const=0  gui_display_data_type=Fixed-point  arith_type=Unsigned  n_bits=1  bin_pt=0  preci_type=Single  exp_width=8  frac_width=24  explicit_period=off  period=1  equ=P=C  opselect=C  inp2=PCIN>>17  opr=+  inp1=P  carry=CIN  dbl_ovrd=off  block_type=constant
  carryinsel{0..3} (4 alike) : xbsIndex_r4/Constant  const=0  gui_display_data_type=Fixed-point  arith_type=Unsigned  n_bits=3  bin_pt=0  preci_type=Single  exp_width=8  frac_width=24  explicit_period=off  period=1  equ=P=C  opselect=C  inp2=PCIN>>17  opr=+  inp1=P  carry=CIN  dbl_ovrd=off  block_type=constant
  cast_c_im : xbsIndex_r4/Convert  gui_display_data_type=Fixed-point  arith_type="Signed  (2's comp)"  n_bits=9  bin_pt=6  float_type=Single  exp_bits=8  fraction_bits=24  quantization=Truncate  overflow=Wrap  en=off  latency=0  dbl_ovrd=off  pipeline=on  block_type=convert
  cast_c_re : xbsIndex_r4/Convert  gui_display_data_type=Fixed-point  arith_type="Signed  (2's comp)"  n_bits=9  bin_pt=6  float_type=Single  exp_bits=8  fraction_bits=24  quantization=Truncate  overflow=Wrap  en=off  latency=0  dbl_ovrd=off  pipeline=on  block_type=convert
  opmode0 : xbsIndex_r4/Constant  const=5  gui_display_data_type=Fixed-point  arith_type=Unsigned  n_bits=7  bin_pt=0  preci_type=Single  exp_width=8  frac_width=24  explicit_period=off  period=1  equ=P=C  opselect=C  inp2=PCIN>>17  opr=+  inp1=P  carry=CIN  dbl_ovrd=off  block_type=constant
  opmode1 : xbsIndex_r4/Constant  const=21  gui_display_data_type=Fixed-point  arith_type=Unsigned  n_bits=7  bin_pt=0  preci_type=Single  exp_width=8  frac_width=24  explicit_period=off  period=1  equ=P=C  opselect=C  inp2=PCIN>>17  opr=+  inp1=P  carry=CIN  dbl_ovrd=off  block_type=constant
  opmode2 : xbsIndex_r4/Constant  const=5  gui_display_data_type=Fixed-point  arith_type=Unsigned  n_bits=7  bin_pt=0  preci_type=Single  exp_width=8  frac_width=24  explicit_period=off  period=1  equ=P=C  opselect=C  inp2=PCIN>>17  opr=+  inp1=P  carry=CIN  dbl_ovrd=off  block_type=constant
  opmode3 : xbsIndex_r4/Constant  const=21  gui_display_data_type=Fixed-point  arith_type=Unsigned  n_bits=7  bin_pt=0  preci_type=Single  exp_width=8  frac_width=24  explicit_period=off  period=1  equ=P=C  opselect=C  inp2=PCIN>>17  opr=+  inp1=P  carry=CIN  dbl_ovrd=off  block_type=constant
  realign_a_im : xbsIndex_r4/Convert  gui_display_data_type=Fixed-point  arith_type="Signed  (2's comp)"  n_bits=4  bin_pt=3  float_type=Single  exp_bits=8  fraction_bits=24  quantization=Truncate  overflow=Wrap  en=off  latency=0  dbl_ovrd=off  pipeline=on  block_type=convert
  realign_a_re : xbsIndex_r4/Convert  gui_display_data_type=Fixed-point  arith_type="Signed  (2's comp)"  n_bits=4  bin_pt=3  float_type=Single  exp_bits=8  fraction_bits=24  quantization=Truncate  overflow=Wrap  en=off  latency=0  dbl_ovrd=off  pipeline=on  block_type=convert
  realign_b_im : xbsIndex_r4/Convert  gui_display_data_type=Fixed-point  arith_type="Signed  (2's comp)"  n_bits=4  bin_pt=3  float_type=Single  exp_bits=8  fraction_bits=24  quantization=Truncate  overflow=Wrap  en=off  latency=0  dbl_ovrd=off  pipeline=on  block_type=convert
  realign_b_re : xbsIndex_r4/Convert  gui_display_data_type=Fixed-point  arith_type="Signed  (2's comp)"  n_bits=4  bin_pt=3  float_type=Single  exp_bits=8  fraction_bits=24  quantization=Truncate  overflow=Wrap  en=off  latency=0  dbl_ovrd=off  pipeline=on  block_type=convert
  reinterp_a_im : xbsIndex_r4/Reinterpret  force_arith_type=on  arith_type="Signed  (2's comp)"  force_bin_pt=on  bin_pt=0  block_type=reinterpret
  reinterp_a_re : xbsIndex_r4/Reinterpret  force_arith_type=on  arith_type="Signed  (2's comp)"  force_bin_pt=on  bin_pt=0  block_type=reinterpret
  reinterp_b_im : xbsIndex_r4/Reinterpret  force_arith_type=on  arith_type="Signed  (2's comp)"  force_bin_pt=on  bin_pt=0  block_type=reinterpret
  reinterp_b_re : xbsIndex_r4/Reinterpret  force_arith_type=on  arith_type="Signed  (2's comp)"  force_bin_pt=on  bin_pt=0  block_type=reinterpret
  reinterp_c_im : xbsIndex_r4/Reinterpret  force_arith_type=on  arith_type="Signed  (2's comp)"  force_bin_pt=on  bin_pt=6  block_type=reinterpret
  reinterp_c_re : xbsIndex_r4/Reinterpret  force_arith_type=on  arith_type="Signed  (2's comp)"  force_bin_pt=on  bin_pt=6  block_type=reinterpret
  c_re : Outport
  c_im : Outport  Port=2
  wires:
  b_im/1 -> realign_b_im/1
  b_re/1 -> realign_b_re/1
  a_im/1 -> realign_a_im/1
  a_re/1 -> realign_a_re/1
  cast_c_im/1 -> c_im/1
  cast_c_re/1 -> c_re/1
  reinterp_b_im/1 -> Convert3/1, Convert7/1
  reinterp_b_re/1 -> Convert6/1, Convert4/1
  reinterp_a_im/1 -> Convert/1, Convert1/1
  reinterp_a_re/1 -> Convert5/1, Convert2/1
  realign_b_im/1 -> reinterp_b_im/1
  realign_b_re/1 -> reinterp_b_re/1
  realign_a_im/1 -> reinterp_a_im/1
  realign_a_re/1 -> reinterp_a_re/1
  Convert/1 -> DSP48E_3/1
  DSP48E_2/1 -> Terminator/1
  DSP48E_2/2 -> DSP48E_3/3
  opmode3/1 -> DSP48E_3/4
  alumode3/1 -> DSP48E_3/5
  carryin3/1 -> DSP48E_3/6
  carryinsel3/1 -> DSP48E_3/7
  Convert3/1 -> DSP48E_3/2
  Convert2/1 -> DSP48E_2/1
  Convert4/1 -> DSP48E_2/2
  opmode2/1 -> DSP48E_2/3
  alumode2/1 -> DSP48E_2/4
  carryin2/1 -> DSP48E_2/5
  carryinsel2/1 -> DSP48E_2/6
  reinterp_c_re/1 -> cast_c_re/1
  DSP48E_3/1 -> reinterp_c_re/1
  Convert1/1 -> DSP48E_1/1
  DSP48E_0/1 -> Terminator1/1
  DSP48E_0/2 -> DSP48E_1/3
  opmode1/1 -> DSP48E_1/4
  alumode1/1 -> DSP48E_1/5
  carryin1/1 -> DSP48E_1/6
  carryinsel1/1 -> DSP48E_1/7
  Convert6/1 -> DSP48E_1/2
  Convert5/1 -> DSP48E_0/1
  Convert7/1 -> DSP48E_0/2
  opmode0/1 -> DSP48E_0/3
  alumode0/1 -> DSP48E_0/4
  carryin0/1 -> DSP48E_0/5
  carryinsel0/1 -> DSP48E_0/6
  DSP48E_1/1 -> reinterp_c_im/1
  reinterp_c_im/1 -> cast_c_im/1

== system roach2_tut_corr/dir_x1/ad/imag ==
  addr : Inport
  data_in : Inport  Port=2
  we : Inport  Port=3
  calc_add : Subsystem
  convert_addr : xbsIndex_r4/Convert  gui_display_data_type=Fixed-point  arith_type=Unsigned  n_bits=addr_width  bin_pt=0  float_type=Single  exp_bits=8  fraction_bits=24  quantization=Truncate  overflow=Wrap  en=off  latency=0  dbl_ovrd=off  pipeline=off  block_type=convert
  convert_din1 : xbsIndex_r4/Convert  gui_display_data_type=Fixed-point  arith_type=Unsigned  n_bits=32  bin_pt=0  float_type=Single  exp_bits=8  fraction_bits=24  quantization=Truncate  overflow=Wrap  en=off  latency=0  dbl_ovrd=off  pipeline=off  block_type=convert
  convert_we : xbsIndex_r4/Convert  gui_display_data_type=Fixed-point  arith_type=Unsigned  n_bits=1  bin_pt=0  float_type=Single  exp_bits=8  fraction_bits=24  quantization=Truncate  overflow=Wrap  en=off  latency=0  dbl_ovrd=off  pipeline=off  block_type=convert
  mem : Subsystem
  munge_in : Subsystem  AncestorBlock=casper_library_flow_control/munge
  munge_out : Subsystem  AncestorBlock=casper_library_flow_control/munge
  roach2_tut_corr_dir_x1_ad_imag_addr : xbsIndex_r4/Gateway Out  inherit_from_input=off  hdl_port=on  timing_constraint=None  locs_specified=off  LOCs={'A5','B9','A9','C1','A3','G6','E9','A6','A7','A8','B8','B1','B3','D9','B5','B4','B6','C2'}  UseAsDAC=off  DACChannel='1'  block_type=gatewayout
  roach2_tut_corr_dir_x1_ad_imag_data_in : xbsIndex_r4/Gateway Out  inherit_from_input=off  hdl_port=on  timing_constraint=None  locs_specified=off  LOCs={'B21','B22','A22','B23','B19','C19','A20','A21','A23','B24','A24','A25','E18','D18','C18','B18'}  UseAsDAC=off  DACChannel='1'  block_type=gatewayout
  roach2_tut_corr_dir_x1_ad_imag_data_out : xbsIndex_r4/Gateway In  gui_display_data_type=Fixed-point  arith_type=Unsigned  n_bits=32  bin_pt=0  preci_type=Single  exp_width=8  frac_width=24  quantization=Truncate  overflow=Wrap  period=sample_rate  dbl_ovrd=off  timing_constraint=None  locs_specified=off  LOCs={}  UseAsADC=off  ADCChannel='1'  inherit_from_input=off  hdl_port=on  block_type=gatewayin
  roach2_tut_corr_dir_x1_ad_imag_we : xbsIndex_r4/Gateway Out  inherit_from_input=off  hdl_port=on  timing_constraint=None  locs_specified=off  LOCs={'A14'}  UseAsDAC=off  DACChannel='1'  block_type=gatewayout
  data_out : Outport
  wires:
  convert_addr/1 -> roach2_tut_corr_dir_x1_ad_imag_addr/1
  convert_din1/1 -> roach2_tut_corr_dir_x1_ad_imag_data_in/1
  data_in/1 -> munge_in/1(din)
  calc_add/1(out) -> convert_addr/1
  roach2_tut_corr_dir_x1_ad_imag_we/1 -> mem/3(In3)
  roach2_tut_corr_dir_x1_ad_imag_data_in/1 -> mem/2(In2)
  roach2_tut_corr_dir_x1_ad_imag_addr/1 -> mem/1(In1)
  convert_we/1 -> roach2_tut_corr_dir_x1_ad_imag_we/1
  roach2_tut_corr_dir_x1_ad_imag_data_out/1 -> munge_out/1(din)
  mem/1(Out1) -> roach2_tut_corr_dir_x1_ad_imag_data_out/1
  addr/1 -> calc_add/1(in)
  we/1 -> convert_we/1
  munge_out/1(dout) -> data_out/1
  munge_in/1(dout) -> convert_din1/1
